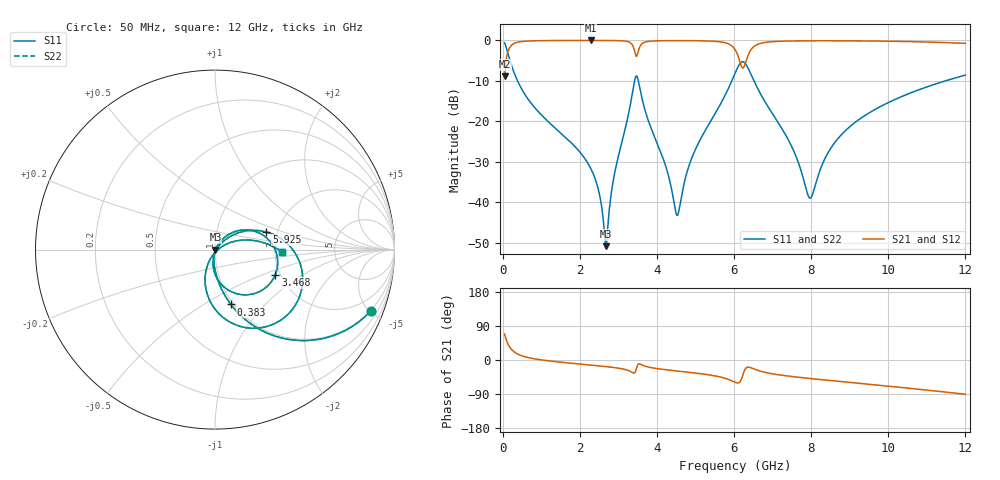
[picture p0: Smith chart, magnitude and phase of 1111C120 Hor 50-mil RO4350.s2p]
# GHz S MA R 50
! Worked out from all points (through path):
!   11951 points, 50 MHz to 12 GHz, reference 50 ohm
!   highest |S21| = -0.02 dB at 2.278 GHz (marker M1); lowest = -8.9 dB at 50 MHz (marker M2)
!   group delay of S21, straight-line fit = 22 ps
!   lowest |S11| = -50.8 dB at 2.678 GHz (marker M3), VSWR 1.01, Z = 50.3 - j0.101 ohm
!   |S11| at or under -10 dB: 385 MHz to 3.42 GHz (3.035 GHz wide, 160 % of centre); 3.519 GHz to 5.942 GHz (2.424 GHz wide, 51.2 % of centre); 6.516 GHz to 11.48 GHz (4.964 GHz wide, 55.2 % of centre)
!   |S22| runs from -50.8 to -0.6 dB; largest |S21 - S12| = 0
!   S11 on the Smith chart (normalised r, x): 50 MHz: 0.97, -5.10; 383 MHz: 0.97, -0.66; 3.468 GHz: 1.88, -0.61; 5.925 GHz: 1.75, +0.38; 12 GHz: 2.19, -0.06
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0.05  0.9328 -21.4  0.3602 68.6  0.3602 68.6  0.9328 -21.4
0.205  0.533 -59.1  0.8457 30.9  0.8457 30.9  0.533 -59.1
0.383  0.3178 -73.9  0.9475 16.0  0.9475 16.0  0.3178 -73.9
2.042  0.03952 -98.9  0.9976 -11.0  0.9976 -11.0  0.03952 -98.9
2.278  0.0265 -99.5  0.9977 -13.3  0.9977 -13.3  0.0265 -99.5
2.678  0.002877 -20.4  0.997 -17.4  0.997 -17.4  0.002877 -20.4
2.901  0.02258 57.5  0.9947 -20.1  0.9947 -20.1  0.02258 57.5
3.347  0.1999 33.3  0.9 -32.1  0.9 -32.1  0.1999 33.3
3.468  0.3641 -22.7  0.6357 -22.2  0.6357 -22.2  0.3641 -22.7
3.641  0.1692 -84.5  0.9296 -14.3  0.9296 -14.3  0.1692 -84.5
4.034  0.04995 -100.8  0.9879 -23.1  0.9879 -23.1  0.04995 -100.8
4.536  0.006945 -21.4  0.9929 -29.1  0.9929 -29.1  0.006945 -21.4
4.937  0.03858 44.7  0.9912 -33.6  0.9912 -33.6  0.03858 44.7
5.925  0.3028 18.9  0.8685 -54.1  0.8685 -54.1  0.3028 18.9
6.025  0.3905 6.8  0.7726 -58.7  0.7726 -58.7  0.3905 6.8
6.178  0.5321 -25.1  0.4986 -53.3  0.4986 -53.3  0.5321 -25.1
6.332  0.4844 -64.7  0.5974 -19.5  0.5974 -19.5  0.4844 -64.7
6.66  0.2306 -102.3  0.9098 -28.7  0.9098 -28.7  0.2306 -102.3
8.017  0.01193 -26.7  0.9886 -49.3  0.9886 -49.3  0.01193 -26.7
8.679  0.06007 25.4  0.9887 -55.9  0.9887 -55.9  0.06007 25.4
10.009  0.1713 18.2  0.9766 -69.1  0.9766 -69.1  0.1713 18.2
12  0.373 -1.8  0.9187 -90.5  0.9187 -90.5  0.373 -1.8
